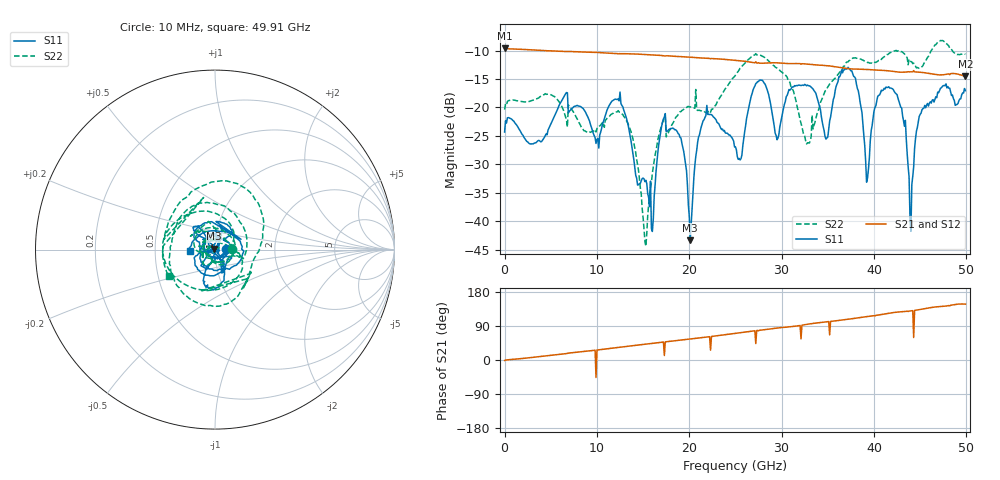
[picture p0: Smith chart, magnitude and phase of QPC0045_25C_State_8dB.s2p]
!File name = QPC0045_25C_State_8dB.s2p
!Date Time: 2024/05/02 05:42:16 AM
!Cal Ref Plane:TRL
!TEMP = 25C
!Vdd(V) = 3.15
!Vss(V) = 0.000
# GHz  S  DB  R  50
!%	Freq(GHz)  S11(dB)  S11(deg)  S21(dB)  S21(deg)  S12(dB)  S12(deg)  S22(dB)  S22(deg)
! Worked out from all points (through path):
!   500 points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, 10 MHz to 49.91 GHz, reference 50 ohm
!   highest |S21| = -9.60 dB at 10 MHz (marker M1); lowest = -14.5 dB at 49.91 GHz (marker M2)
!   lowest |S11| = -43.4 dB at 20.11 GHz (marker M3), VSWR 1.01, Z = 49.5 + j0.496 ohm
!   |S11| at or under -10 dB: start of sweep to end of sweep
!   |S22| runs from -44.4 to -8.2 dB; largest |S21 - S12| = 0.0011
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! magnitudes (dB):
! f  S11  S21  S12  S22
! 10 MHz  -24.3  -9.6  -9.6  -20.4
! 8.41 GHz  -20.1  -10.2  -10.2  -23.7
! 13.01 GHz  -20.9  -10.6  -10.5  -21.8
! 15.21 GHz  -33.0  -10.7  -10.7  -43.6
! 16.11 GHz  -39.7  -10.8  -10.8  -30.4
! 16.71 GHz  -26.4  -10.8  -10.8  -24.9
! 18.91 GHz  -24.7  -11.1  -11.0  -21.0
! 20.11 GHz  -43.4  -11.2  -11.2  -19.9
! 21.71 GHz  -21.7  -11.3  -11.3  -20.8
! 25.01 GHz  -26.9  -11.7  -11.7  -14.3
! 27.41 GHz  -15.5  -12.2  -12.2  -10.7
! 29.51 GHz  -25.7  -12.2  -12.1  -13.1
! 33.31 GHz  -16.6  -12.4  -12.4  -21.3
! 34.91 GHz  -25.4  -12.7  -12.7  -16.7
! 37.51 GHz  -13.5  -13.2  -13.2  -11.5
! 39.31 GHz  -32.4  -13.3  -13.3  -12.1
! 40.21 GHz  -19.7  -13.4  -13.4  -12.1
! 41.61 GHz  -16.4  -13.6  -13.6  -10.5
! 43.21 GHz  -22.3  -13.8  -13.8  -10.4
! 44.01 GHz  -41.8  -13.7  -13.7  -11.9
! 45.11 GHz  -21.0  -13.8  -13.8  -13.0
! 49.91 GHz  -17.0  -14.5  -14.5  -10.7
